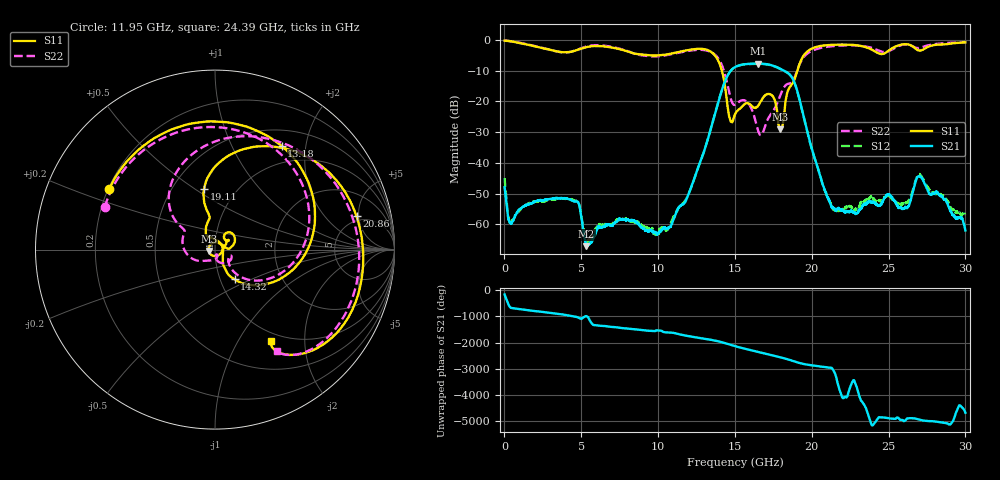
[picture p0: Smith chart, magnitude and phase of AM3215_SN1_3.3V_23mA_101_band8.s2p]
!Agilent Technologies,E8364B,MY43040894,A.07.50.67
!Agilent E8364B: A.07.50.67
!Date: Tuesday, May 25, 2021 15:31:33
!Correction: S11(Full 2 Port(1,2))
!S21(Full 2 Port(1,2))
!S12(Full 2 Port(1,2))
!S22(Full 2 Port(1,2))
!S2P File: Measurements: S11, S21, S12, S22:
# Hz S  dB  R 50
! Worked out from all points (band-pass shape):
!   6401 points, 10 MHz to 30 GHz, reference 50 ohm
!   highest |S21| = -7.73 dB at 16.51 GHz (marker M1); lowest = -67.1 dB at 5.333 GHz (marker M2)
!   |S21| within 3 dB of the highest: 14.63 GHz to 18.44 GHz (3.806 GHz wide, 23 % of centre)
!   lowest |S11| = -29.1 dB at 17.95 GHz (marker M3), VSWR 1.07, Z = 46.7 - j0.646 ohm
!   |S11| at or under -10 dB: 14.15 GHz to 19.07 GHz (4.917 GHz wide, 29.6 % of centre)
!   |S22| runs from -31.0 to -0.2 dB; largest |S21 - S12| = 0.0081
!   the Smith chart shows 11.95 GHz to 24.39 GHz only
!   S11 on the Smith chart (normalised r, x): 11.95 GHz: 0.20, +0.26; 13.18 GHz: 0.73, +1.59; 14.32 GHz: 1.17, -0.40; 19.11 GHz: 0.71, +0.55; 20.86 GHz: 4.34, +4.69; 24.39 GHz: 0.88, -1.38
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1e7  -0.32 -6.3  -47.94 -164.0  -44.97 -57.9  -0.23 -6.4
9.753031e8  -1.03 -85.0  -55.06 -0.8  -55.57 -1.5  -0.95 -84.1
2.104614e9  -2.30 -167.5  -52.41 -84.8  -52.50 -83.1  -2.20 -165.4
3.566627e9  -3.92 79.2  -51.47 171.9  -51.54 170.3  -3.96 84.5
5.009895e9  -2.88 -71.9  -57.74 -16.9  -57.49 67.0  -2.73 -64.8
5.333225e9  -2.41 -102.7  -67.09 90.3  -65.55 64.0  -2.20 -95.6
6.33133e9  -2.09 178.3  -60.86 76.8  -60.29 171.8  -1.84 -173.8
7.549673e9  -3.12 100.3  -58.52 -0.5  -58.69 2.7  -2.97 108.4
1.000979e10  -5.10 -69.0  -62.76 -101.2  -63.10 -77.4  -5.38 -65.6
1.194508e10  -3.35 150.0  -50.64 48.1  -50.60 51.1  -3.63 158.8
1.317748e10  -3.27 57.2  -33.37 -71.1  -33.36 -70.0  -3.53 69.5
1.432085e10  -14.06 -56.6  -13.94 141.7  -13.89 141.2  -10.74 -36.5
1.5005e10  -24.24 22.2  -8.89 20.6  -8.91 20.3  -21.16 -25.4
1.574538e10  -20.65 35.2  -7.90 -91.8  -7.97 -92.0  -19.99 -45.5
1.651387e10  -21.32 54.1  -7.73 161.9  -7.82 162.1  -29.65 -84.1
1.795245e10  -29.15 -168.6  -9.43 -45.1  -9.50 -44.5  -17.97 -153.2
1.911457e10  -9.26 100.2  -17.68 110.3  -17.83 111.3  -9.14 136.6
2.00049e10  -2.87 47.6  -35.38 8.2  -35.53 10.0  -3.62 73.3
2.085774e10  -1.83 13.3  -48.92 -61.8  -49.11 -60.0  -2.40 31.8
2.438625e10  -4.50 -58.7  -53.78 179.3  -52.38 172.9  -3.58 -58.8
2.500479e10  -3.55 -51.9  -50.35 143.4  -50.39 144.6  -3.70 -56.7
3e10  -0.84 -109.1  -61.97 -9.6  -56.57 178.3  -0.75 -112.4
